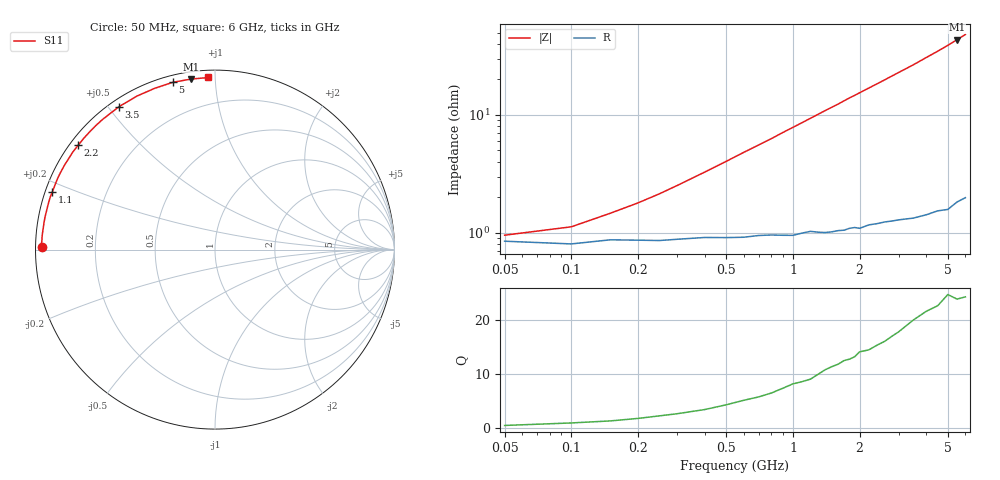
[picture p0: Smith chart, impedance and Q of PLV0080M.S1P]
! Infineon Technologies  Discrete & RF Semiconductors
! BAR 64-04W /-05W /-06W
! Si PIN Diode in SOT323
! IF = 80 mA
! S-Parameters:  October  2008
# GHz  S  MA  R  50
!  f  S11
! GHz  MAG  ANG
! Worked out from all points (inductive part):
!   34 points, 50 MHz to 6 GHz, reference 50 ohm
!   read as one part to ground: L = 1.25 nH near 400 MHz
!   highest Q = 24.2 at 5.5 GHz (marker M1), where L = 1.26 nH
!   S11 on the Smith chart (normalised r, x): 50 MHz: 0.02, +0.01; 1.1 GHz: 0.02, +0.17; 2.2 GHz: 0.02, +0.34; 3.5 GHz: 0.03, +0.53; 5 GHz: 0.03, +0.78; 6 GHz: 0.04, +0.96
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0.05  0.9666 179.0
0.1  0.9683 178.2
0.15  0.9657 177.3
0.25  0.9662 175.5
0.5  0.9645 171.0
0.6  0.9643 169.2
0.8  0.9629 165.8
0.9  0.9633 164.0
1  0.9635 162.3
1.1  0.9621 160.6
1.2  0.961 158.9
1.4  0.9623 155.5
1.6  0.9614 152.3
1.7  0.9614 150.6
1.8  0.9603 148.9
1.9  0.96 147.4
2  0.9609 145.8
2.2  0.9589 142.7
2.4  0.9587 139.7
2.6  0.9582 136.7
2.8  0.9583 133.7
3  0.9583 130.8
3.5  0.9593 123.9
4  0.9595 116.9
4.5  0.9594 110.5
5  0.9614 104.2
5.5  0.9593 98.0
6  0.9596 92.2
